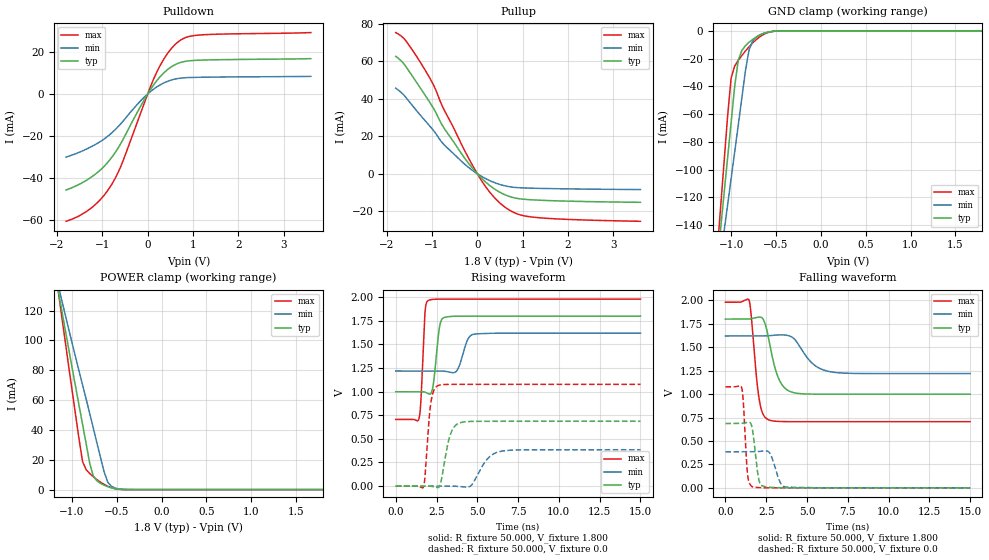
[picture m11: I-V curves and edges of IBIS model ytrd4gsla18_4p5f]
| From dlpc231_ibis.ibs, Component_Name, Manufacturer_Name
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| Model ytrd4gsla18_4p5f
[Model] ytrd4gsla18_4p5f
Model_type 3-state
Polarity   Non-Inverting
Enable   Active-High
Vmeas =  0.900V
Cref =  50.000pF
Rref =  0.500k
Vref =  0.0V
C_comp   1.982pF   1.912pF   2.009pF
C_comp_pullup   1.007pF   0.932pF   1.068pF
C_comp_pulldown   1.007pF   0.932pF   1.068pF
[Temperature Range]   25.000   0.125k   -40.000
[Voltage Range]   1.800V   1.620V   1.980V
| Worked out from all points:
|   slope of the pulldown table from 0 to 0.27 V, typ, clamps not added: 33.2 ohm
|   slope of the pullup table from 0 to 0.27 V, typ, clamps not added: 43.8 ohm
|   GND clamp passes 1 mA (typ) near -0.59 V on its own axis
|   POWER clamp passes 1 mA (typ) near -0.54 V on its own axis
|   rising waveform, R_fixture 50.000, V_fixture 1.800: 20-80 % time 281ps typ, 430ps min, 193ps max; typ from 0.999 V to 1.8 V
|   rising waveform, R_fixture 50.000, V_fixture 0.0: 20-80 % time 482ps typ, 842ps min, 297ps max; typ from 0 V to 0.686 V
|   falling waveform, R_fixture 50.000, V_fixture 1.800: 20-80 % time 685ps typ, 1.1ns min, 415ps max; typ from 1.8 V to 0.999 V
|   falling waveform, R_fixture 50.000, V_fixture 0.0: 20-80 % time 279ps typ, 425ps min, 203ps max; typ from 0.686 V to 0 V
[Pulldown]
-1.8V     -45.9mA    -30.16mA   -60.85mA
-1.2V     -39.06mA   -24.69mA   -53.7mA
-960mV    -34.59mA   -21.53mA   -48.4mA
-780mV    -29.93mA   -18.34mA   -42.75mA
-540mV    -21.58mA   -12.91mA   -31.78mA
-120mV    -4.493mA   -2.485mA   -7.075mA
180mV     5.802mA    3.075mA    9.47mA
420mV     11.33mA    5.896mA    18.81mA
660mV     14.57mA    7.386mA    24.71mA
840mV     15.65mA    7.797mA    27.01mA
1.14V     16.17mA    7.999mA    28.19mA
3.6V      16.91mA    8.437mA    29.37mA
[Pullup]
-1.8V     62.53mA    45.59mA    75.18mA
-1.56V    56.51mA    40.18mA    70.26mA
-1.08V    39.2mA     26.26mA    52.3mA
-960mV    34.6mA     22.86mA    46.95mA
-720mV    23.8mA     15.14mA    33.46mA
-180mV    5.162mA    3.128mA    7.765mA
60mV      -1.548mA   -908uA     -2.405mA
240mV     -5.585mA   -3.264mA   -8.722mA
600mV     -11.07mA   -6.366mA   -17.6mA
900mV     -13.21mA   -7.4mA     -21.53mA
1.26V     -13.94mA   -7.707mA   -23.17mA
3.6V      -15.2mA    -8.399mA   -25.3mA
[GND_clamp]
-1.8V     -597.4mA   -500.9mA   -710mA
-1.16V    -170.9mA   -184.3mA   -163.5mA
-1.12V    -144.6mA   -164.8mA   -129.7mA
-1.08V    -118.4mA   -145.4mA   -95.95mA
-1.04V    -92.22mA   -126mA     -62.27mA
-1V       -66.09mA   -106.6mA   -34.11mA
-960mV    -39.93mA   -87.3mA    -25.33mA
-920mV    -21.05mA   -67.84mA   -21.23mA
-800mV    -8.254mA   -13.78mA   -11.5mA
-680mV    -3.146mA   -2.862mA   -4.259mA
-440mV    -43.6uA    -64.31uA   -34.79uA
1.8V      0A         0A         0A
[POWER_clamp]
-1.8V     367.9mA    313.2mA    432.7mA
-1.16V    136.5mA    139.2mA    137mA
-1.12V    123mA      129mA      119.6mA
-920mV    56.74mA    79.65mA    34.28mA
-880mV    43.81mA    70.18mA    18.86mA
-840mV    30.81mA    60.69mA    13.38mA
-800mV    17.64mA    50.99mA    10.77mA
-760mV    9.019mA    41.18mA    8.633mA
-680mV    4.212mA    21.63mA    4.996mA
-600mV    1.988mA    5.044mA    2.281mA
-480mV    292.3uA    521.1uA    246.1uA
1.8V      0A         0A         0A
[Ramp]
dV/dt_r 0.412/0.481n   0.231/0.851n   0.647/0.298n
dV/dt_f 0.481/0.689n   0.241/1.100n   0.764/0.416n
R_load = 50.000
[Rising Waveform]
R_fixture= 50.000
V_fixture= 1.800
V_fixture_min= 1.620
V_fixture_max= 1.980
0s        999.1mV    1.219V     706.3mV
1.428ns   999.4mV    1.219V     715.9mV
1.548ns   999.5mV    1.219V     921.3mV
1.798ns   994.4mV    1.219V     1.848V
2.008ns   976.9mV    1.219V     1.967V
2.258ns   1.033V     1.219V     1.977V
2.979ns   1.786V     1.217V     1.98V
3.739ns   1.799V     1.221V     1.98V
4.791ns   1.8V       1.608V     1.98V
15ns      1.8V       1.62V      1.98V
[Rising Waveform]
R_fixture= 50.000
V_fixture= 0.0
V_fixture_min= 0.0
V_fixture_max= 0.0
0s        0V         0V         0V
1.698ns   135.3uV    0V         -10.24mV
2.147ns   -1.234mV   -3.661uV   874.4mV
2.599ns   -15.95mV   -2.092uV   1.064V
3.329ns   535.2mV    343.6uV    1.077V
3.918ns   669.1mV    -5.096mV   1.078V
4.617ns   684.7mV    5.113mV    1.078V
5.578ns   686.2mV    280mV      1.078V
6.398ns   686.3mV    366.6mV    1.078V
15ns      686.3mV    384.6mV    1.078V
[Falling Waveform]
R_fixture= 50.000
V_fixture= 1.800
V_fixture_min= 1.620
V_fixture_max= 1.980
0s        1.8V       1.62V      1.98V
1.449ns   1.8V       1.62V      2.002V
2.069ns   1.821V     1.62V      946.3mV
2.359ns   1.784V     1.62V      769.5mV
2.629ns   1.611V     1.621V     727.5mV
3.259ns   1.168V     1.631V     708.4mV
4.109ns   1.019V     1.605V     706.4mV
5.319ns   1V         1.329V     706.3mV
6.429ns   999.2mV    1.239V     706.3mV
15ns      999.1mV    1.219V     706.3mV
[Falling Waveform]
R_fixture= 50.000
V_fixture= 0.0
V_fixture_min= 0.0
V_fixture_max= 0.0
0s        686.3mV    384.6mV    1.078V
999ps     687.7mV    384.4mV    1.068V
1.099ns   689.3mV    384.4mV    915.4mV
1.349ns   698.8mV    384.5mV    160.6mV
1.648ns   630.3mV    385.1mV    12.08mV
2.039ns   97.6mV     388.2mV    2.946mV
2.409ns   13.26mV    394.8mV    752.9uV
2.747ns   5.904mV    363.4mV    207.2uV
3.648ns   672.4uV    10.67mV    6.37uV
15ns      0V         0V         0V
